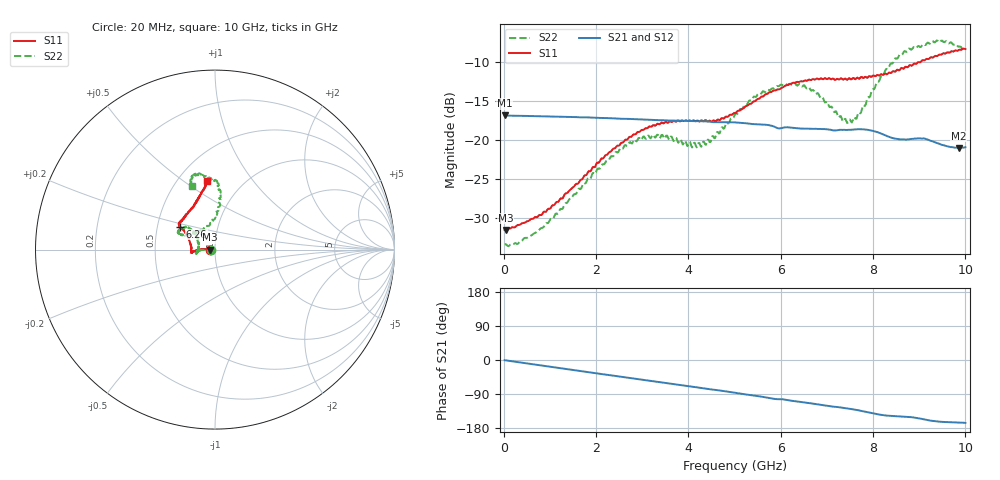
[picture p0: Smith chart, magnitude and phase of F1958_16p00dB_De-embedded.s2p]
! Integrated Device Technology
! Corporate Headquarters
! 6024 Silver Creek Valley Road
! San Jose, CA 95138  USA
! Phone:  1-408-284-8200
! Toll Free:  1-800-223-1366
! Webpage:  http://www.idt.com/
! Timing and RF Division
! 515 Groton Road, Suite 102
! Westford, MA 01886-6024
! Device:  F1958
! Description: 7-bit 0.25 dB Digital Step Attenuator
! Frequency:  0.001 -  6.000 GHz
! Package:  4x4 mm Thin QFN Plastic Package: 24 pin
! Ports:  2 RF, 12 DC
!  Pin  1  = D0
!  Pin  2  = VDD
!  Pin  3  = VMODE
!  Pin  4  = GND
!  Pin  5  = RF1  =  Port 1
!  Pin  6  = GND
!  Pin  7  = GND
!  Pin  8  = GND
!  Pin  9  = GND
!  Pin 10  = GND
!  Pin 11  = GND
!  Pin 12  = GND
!  Pin 13  = GND
!  Pin 14  = RF2  =  Port 2
!  Pin 15  = GND
!  Pin 16  = LE
!  Pin 17  = CLK
!  Pin 18  = DATA
!  Pin 19  = D6
!  Pin 20  = D5
!  Pin 21  = D4
!  Pin 22  = D3
!  Pin 23  = D2
!  Pin 24  = D1
! State:  64
! Atten State:  16.00 dB
! Voltage:  +3.30 Volts
! Current:  0.258 mA
! Data:  The device was measured on a F1958 evaluation board which has
!  individual transmission lines to the RF pins.  Data was collected
!  using a calibrated network analyzer.  The evaluation board was
!  de-embedded using Automatic Fixture Removal (AFR).
!  The reference plane is the edge of the package pin.
! Misc:
!  Action Tracker AT0419
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# GHz S dB R 50
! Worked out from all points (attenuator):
!   500 points, 20 MHz to 10 GHz, reference 50 ohm
!   highest |S21| = -16.84 dB at 20 MHz (marker M1); lowest = -21.0 dB at 9.86 GHz (marker M2)
!   lowest |S11| = -31.6 dB at 40 MHz (marker M3), VSWR 1.05, Z = 47.4 - j0.0749 ohm
!   |S11| at or under -10 dB: start of sweep to 8.973 GHz
!   |S22| runs from -33.7 to -7.2 dB; largest |S21 - S12| = 0.00051
!   S11 on the Smith chart (normalised r, x): 20 MHz: 0.95, -0.00; 6.26 GHz: 0.65, +0.18; 10 GHz: 0.69, +0.62
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0.02  -31.55 -178.2  -16.84 -0.5  -16.83 -0.4  -33.45 -178.3
0.04  -31.58 -178.3  -16.84 -0.8  -16.84 -0.8  -33.39 -177.3
0.32  -30.92 177.5  -16.88 -5.8  -16.88 -5.8  -33.27 177.5
0.84  -29.49 176.0  -16.93 -14.9  -16.93 -14.9  -31.29 178.8
1.7  -25.06 177.5  -17.08 -29.8  -17.07 -29.8  -25.88 178.3
2.62  -20.04 -178.2  -17.27 -45.6  -17.25 -45.6  -20.67 -175.2
2.92  -18.96 -175.5  -17.33 -50.7  -17.31 -50.8  -19.73 -172.4
3.36  -17.96 -173.0  -17.44 -58.3  -17.44 -58.4  -19.59 -167.6
4.3  -17.49 -178.9  -17.57 -74.2  -17.59 -74.2  -20.56 164.5
4.52  -17.60 175.0  -17.69 -78.1  -17.70 -78.1  -19.49 155.5
5.02  -16.52 161.5  -17.73 -86.6  -17.74 -86.6  -16.60 140.7
5.54  -14.66 151.1  -17.98 -95.9  -17.99 -95.9  -14.04 141.8
6.26  -12.65 146.8  -18.42 -108.0  -18.44 -108.0  -12.94 152.7
6.68  -12.20 144.6  -18.56 -114.8  -18.57 -114.7  -13.62 155.3
7.3  -12.06 138.1  -18.69 -125.3  -18.70 -125.2  -16.91 135.5
7.5  -12.09 135.2  -18.69 -128.9  -18.69 -128.7  -17.36 117.6
7.7  -12.12 131.1  -18.60 -133.2  -18.60 -133.2  -16.44 100.8
8.34  -11.34 116.1  -19.58 -147.2  -19.58 -147.3  -10.69 83.9
8.68  -10.70 109.4  -19.93 -149.5  -19.93 -149.5  -8.55 88.0
9.26  -9.34 101.4  -20.13 -160.3  -20.12 -160.3  -7.39 100.5
9.86  -8.40 96.7  -21.01 -165.0  -21.04 -165.0  -7.99 109.2
10  -8.29 96.6  -20.93 -166.0  -20.96 -166.0  -8.47 109.9
